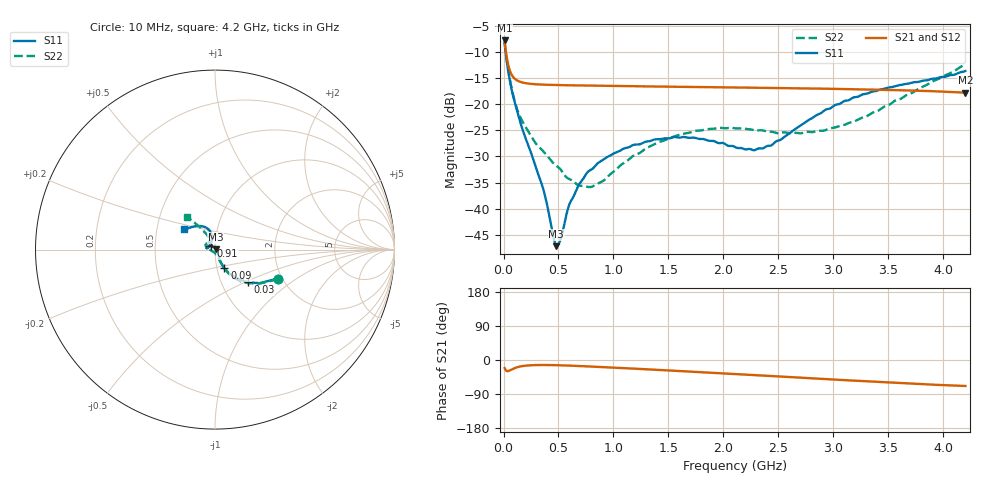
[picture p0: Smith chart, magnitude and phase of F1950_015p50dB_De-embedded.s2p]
! Integrated Device Technology
! Corporate Headquarters
! 6024 Silver Creek Valley Road
! San Jose, CA 95138  USA
! Phone:  1-408-284-8200
! Toll Free:  1-800-223-1366
! Webpage:  http://www.idt.com/
! Timing and RF Division
! 515 Groton Road, Suite 102
! Westford, MA 01886-6024
! Device:  F1950
! Description: 7-bit 0.25 dB Digital Step Attenuator
! Frequency:  150.0 -  4000.00 MHz
! Package:  4x4 mm Thin QFN Plastic Package: 24 pin
! Ports:  2 RF, 12 DC
!  Pin  1  = D0
!  Pin  2  = VDD
!  Pin  3  = Vmode
!  Pin  4  = GND
!  Pin  5  = RF1  =  Port 1
!  Pin  6  = GND
!  Pin  7  = GND
!  Pin  8  = GND
!  Pin  9  = GND
!  Pin 10  = GND
!  Pin 11  = GND
!  Pin 12  = GND
!  Pin 13  = GND
!  Pin 14  = RF2  =  Port 2
!  Pin 15  = GND
!  Pin 16  = LE
!  Pin 17  = CLK
!  Pin 18  = DATE
!  Pin 19  = D6
!  Pin 20  = D5
!  Pin 21  = D4
!  Pin 22  = D3
!  Pin 23  = D2
!  Pin 24  = D1
! State:  62
! Atten State:  15.50 dB
! Voltage:  +5.00 Volts
! Current:  Not Measured mA
! Data:  The device was measured on a the F195X evaluation board which has
!  individual transmission lines to the RF pins.  Data was collected
!  using a calibrated network analyzer.  The evaluation board was
!  de-embedded using a TRL calibration technique.
!  The reference plane is the edge of the package pin.
! Misc:  Board 2019
!  Action Tracker AT0250
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# GHz S dB R 50
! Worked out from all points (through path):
!   420 points, 10 MHz to 4.2 GHz, reference 50 ohm
!   highest |S21| = -7.81 dB at 10 MHz (marker M1); lowest = -17.8 dB at 4.2 GHz (marker M2)
!   group delay of S21, straight-line fit = 39.5 ps
!   lowest |S11| = -47.2 dB at 480 MHz (marker M3), VSWR 1.01, Z = 50.4 + j0.226 ohm
!   |S11| at or under -10 dB: 19.07 MHz to end of sweep
!   |S22| runs from -35.9 to -8.2 dB; largest |S21 - S12| = 0.00022
!   S11 on the Smith chart (normalised r, x): 10 MHz: 1.90, -0.72; 30 MHz: 1.33, -0.52; 90 MHz: 1.08, -0.23; 910 MHz: 0.96, +0.04; 4.2 GHz: 0.69, +0.16
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0.01  -8.26 -24.6  -7.81 -21.2  -7.81 -21.2  -8.22 -25.2
0.03  -11.80 -44.9  -11.10 -29.3  -11.10 -29.3  -11.68 -45.7
0.06  -15.80 -57.8  -13.70 -27.1  -13.70 -27.1  -15.47 -58.7
0.09  -18.67 -63.4  -14.86 -22.8  -14.86 -22.8  -18.48 -62.9
0.15  -23.30 -64.8  -15.71 -17.2  -15.71 -17.2  -22.36 -66.8
0.26  -29.91 -57.5  -16.14 -13.7  -16.14 -13.7  -26.44 -69.0
0.36  -36.17 -44.0  -16.26 -13.2  -16.26 -13.2  -28.99 -72.5
0.45  -44.96 -7.9  -16.32 -13.5  -16.33 -13.5  -31.23 -76.6
0.48  -47.18 30.9  -16.34 -13.7  -16.34 -13.7  -31.78 -80.1
0.52  -45.74 77.3  -16.36 -14.0  -16.36 -14.0  -32.52 -82.0
0.6  -39.09 111.7  -16.39 -14.8  -16.39 -14.8  -34.36 -94.0
0.71  -34.71 125.1  -16.43 -16.1  -16.43 -16.1  -35.63 -113.0
0.91  -30.57 139.4  -16.49 -18.8  -16.49 -18.8  -34.62 -154.7
1.17  -27.90 153.0  -16.57 -22.6  -16.57 -22.6  -30.04 178.5
1.41  -26.72 163.8  -16.63 -26.2  -16.63 -26.2  -27.28 168.2
1.73  -26.41 170.9  -16.71 -31.1  -16.71 -31.1  -25.18 159.1
2.11  -28.25 160.5  -16.81 -37.2  -16.81 -37.2  -24.63 149.6
2.43  -27.93 124.7  -16.90 -42.2  -16.89 -42.2  -25.26 139.7
2.81  -22.63 103.2  -17.01 -48.4  -17.00 -48.4  -25.34 124.4
3.1  -19.37 105.8  -17.11 -53.1  -17.10 -53.2  -23.96 118.9
3.51  -16.78 117.1  -17.28 -59.5  -17.28 -59.5  -20.10 119.4
4.2  -13.65 146.9  -17.79 -68.6  -17.79 -68.7  -12.38 130.3
